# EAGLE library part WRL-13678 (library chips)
ESP8266 WiFi Module https://www.mouser.com/ds/2/813/ESP8266ModuleV1-1095236.pdf
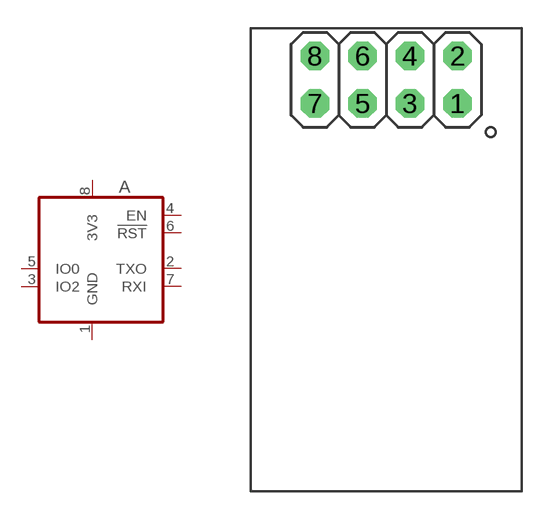
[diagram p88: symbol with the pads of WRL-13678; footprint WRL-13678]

Designator prefix A

## WRL-13678 (DIGIKEY: 1568-1235-ND)  [WRL-13678]
1  GND  pwr
2  TXO
3  IO2
4  EN
5  IO0
6  !RST
7  RXI
8  3V3  pwr

## Footprint WRL-13678 (pad centres in mm)
drill 1.016 octagon: 1 3.81,-1.27; 2 3.81,1.27; 3 1.27,-1.27; 4 1.27,1.27; 5 -1.27,-1.27; 6 -1.27,1.27; 7 -3.81,-1.27; 8 -3.81,1.27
